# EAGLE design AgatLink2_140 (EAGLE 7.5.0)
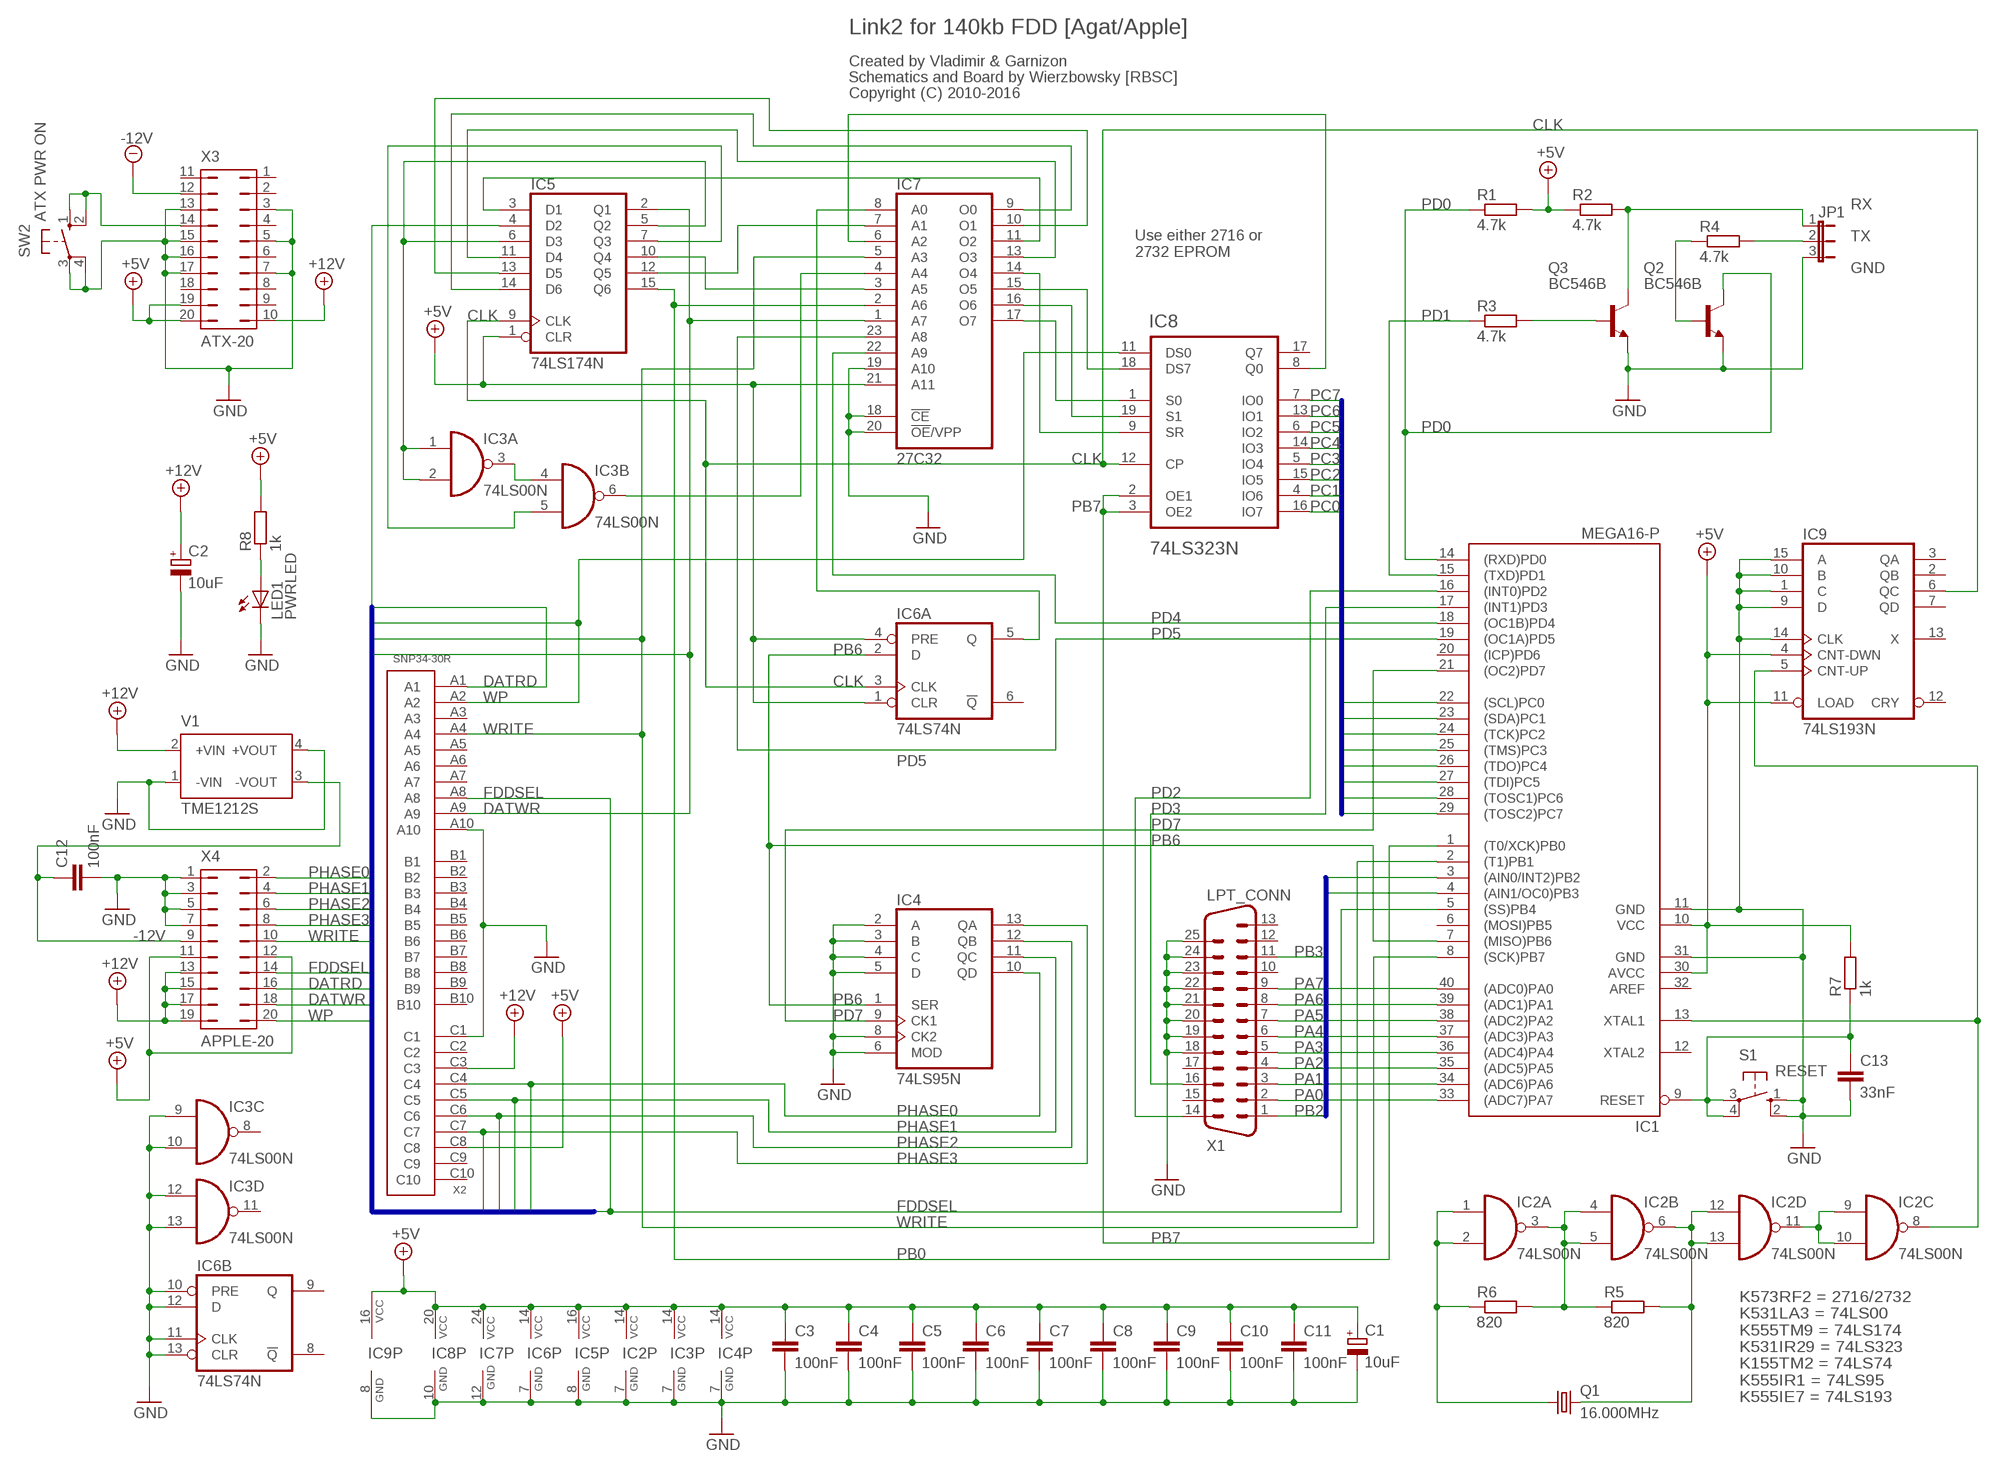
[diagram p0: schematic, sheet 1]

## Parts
C1  10uF  CPOL-EUE2-5  [E2-5]
C2  10uF  CPOL-EUE2-5  [E2-5]
C3  100nF  C-EU050-025X075  [C050-025X075]
C4  100nF  C-EU050-025X075  [C050-025X075]
C5  100nF  C-EU050-025X075  [C050-025X075]
C6  100nF  C-EU050-025X075  [C050-025X075]
C7  100nF  C-EU050-025X075  [C050-025X075]
C8  100nF  C-EU050-025X075  [C050-025X075]
C9  100nF  C-EU050-025X075  [C050-025X075]
C10  100nF  C-EU050-025X075  [C050-025X075]
C11  100nF  C-EU050-025X075  [C050-025X075]
C12  100nF  C-EU050-025X075  [C050-025X075]
C13  33nF  C-EU025-025X050  [C025-025X050]
IC1  MEGA16-P  [DIL40]
IC2  74LS00N  [DIL14]
IC3  74LS00N  [DIL14]
IC4  74LS95N  [DIL14]
IC5  74LS174N  [DIL16]
IC6  74LS74N  [DIL14]
IC7  27C32  2732  [DIL24]
IC8  74LS323N  [DIL20]
IC9  74LS193N  [DIL16]
JP1  JP2E  [JP2]
LED1  PWRLED  LED3MM  [LED3MM]
Q1  16.000MHz  CRYSTALHC49S  [HC49/S]
Q2  BC546B  [TO92-EBC]
Q3  BC546B  [TO92-EBC]
R1  4.7k  R-EU_0204/7  [0204/7]
R2  4.7k  R-EU_0204/7  [0204/7]
R3  4.7k  R-EU_0204/7  [0204/7]
R4  4.7k  R-EU_0204/7  [0204/7]
R5  820  R-EU_0204/7  [0204/7]
R6  820  R-EU_0204/7  [0204/7]
R7  1k  R-EU_0204/7  [0204/7]
R8  1k  R-EU_0204/7  [0204/7]
S1  RESET  10-XX  [B3F-10XX]
SW2  ATX PWR ON  10-XX  [B3F-10XX]
V1  TME1212S  [TME]
X1  LPT_CONN  M25HP  [M25HP]
X2  SNP34-30R  [SNP34-30R]
X3  ATX-20  [ATX-20]
X4  APPLE-20  [APPLE-20]

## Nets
+5V: C1.+ C3.1 C4.1 C5.1 C6.1 C7.1 C8.1 C9.1 C10.1 C11.1 IC1.10(VCC) IC1.30(AVCC) IC2.14(P:VCC) IC3.14(P:VCC) IC4.14(VCC) IC5.1(CLR) IC5.16(VCC) IC6.1(A:CLR) IC6.4(A:PRE) IC6.14(P:VCC) IC7.21(A11) IC7.24(VCC) IC8.20(VCC) IC9.4(CNT-DWN) IC9.11(LOAD) IC9.16(VCC) R1.2 R2.1 R7.2 R8.2 X2.C8 X3.19 X3.20 X4.11 X4.12
+12V: C2.+ V1.2(+VIN) X2.C3 X3.10 X4.13 X4.15 X4.17 X4.19
-12V: C12.1 V1.3(-VOUT) X3.12 X4.9
CLK: IC5.9(CLK) IC6.3(A:CLK) IC8.12(CP) IC9.6(QC)
DATRD: IC5.4(D2) X2.A1 X4.16
DATWR: IC5.2(Q1) IC7.1(A7) X2.A9 X4.18
FDDSEL: IC1.5((SS)PB4) X2.A8 X4.14
GND: C1.- C2.- C3.2 C4.2 C5.2 C6.2 C7.2 C8.2 C9.2 C10.2 C11.2 C12.2 C13.2 IC1.11(GND) IC1.31(GND) IC2.7(P:GND) IC3.7(P:GND) IC3.9(C:I0) IC3.10(C:I1) IC3.12(D:I0) IC3.13(D:I1) IC4.2(A) IC4.3(B) IC4.4(C) IC4.5(D) IC4.6(MOD) IC4.7(GND) IC4.8(CK2) IC5.8(GND) IC6.7(P:GND) IC6.10(B:PRE) IC6.11(B:CLK) IC6.12(B:D) IC6.13(B:CLR) IC7.12(GND) IC7.18(!CE) IC7.19(A10) IC7.20(!OE!/VPP) IC8.10(GND) IC9.1(C) IC9.8(GND) IC9.9(D) IC9.10(B) IC9.14(CLK) IC9.15(A) JP1.3 LED1.K(C) Q2.E Q3.E S1.1(S) S1.2(S1) SW2.3(P) SW2.4(P1) V1.1(-VIN) V1.4(+VOUT) X1.18 X1.19 X1.20 X1.21 X1.22 X1.23 X1.24 X1.25 X2.A10 X2.C1 X3.3 X3.5 X3.7 X3.13 X3.15 X3.16 X3.17 X4.1 X4.3 X4.5 X4.7
N$1: IC2.1(A:I0) IC2.2(A:I1) Q1.1 R6.1
N$2: IC2.3(A:O) IC2.4(B:I0) IC2.5(B:I1) R5.1 R6.2
N$3: IC1.13(XTAL1) IC2.8(C:O) IC9.5(CNT-UP)
N$4: SW2.1(S) SW2.2(S1) X3.14
N$6: IC2.6(B:O) IC2.12(D:I0) IC2.13(D:I1) Q1.2 R5.2
N$8: IC2.9(C:I0) IC2.10(C:I1) IC2.11(D:O)
N$11: C13.1 IC1.9(RESET) R7.1 S1.3(P) S1.4(P1)
N$12: JP1.1 Q3.C R2.2
N$13: Q3.B R3.2
N$15: JP1.2 R4.2
N$16: Q2.B R4.1
N$17: LED1.A R8.1
N$19: IC3.3(A:O) IC3.4(B:I0)
N$20: IC3.1(A:I0) IC3.2(A:I1) IC5.5(Q2) IC5.6(D3)
N$22: IC3.5(B:I1) IC5.7(Q3)
N$23: IC3.6(B:O) IC7.4(A4)
N$24: IC6.5(A:Q) IC7.8(A0)
N$27: IC7.14(O4) IC8.9(SR)
N$28: IC7.17(O7) IC8.1(S0)
N$29: IC7.16(O6) IC8.19(S1)
N$30: IC7.15(O5) IC8.18(DS7)
N$35: IC5.3(D1) IC7.11(O2)
N$36: IC5.11(D4) IC7.13(O3)
N$37: IC5.14(D6) IC7.9(O0)
N$38: IC5.13(D5) IC7.10(O1)
N$39: IC5.10(Q4) IC7.3(A5)
N$40: IC5.12(Q5) IC7.7(A1)
N$41: IC7.6(A2) IC8.8(Q0)
PA0: IC1.40((ADC0)PA0) X1.2
PA1: IC1.39((ADC1)PA1) X1.3
PA2: IC1.38((ADC2)PA2) X1.4
PA3: IC1.37((ADC3)PA3) X1.5
PA4: IC1.36((ADC4)PA4) X1.6
PA5: IC1.35((ADC5)PA5) X1.7
PA6: IC1.34((ADC6)PA6) X1.8
PA7: IC1.33((ADC7)PA7) X1.9
PB0: IC1.1((T0/XCK)PB0) IC5.15(Q6) IC7.2(A6)
PB2: IC1.3((AIN0/INT2)PB2) X1.1
PB3: IC1.4((AIN1/OC0)PB3) X1.11
PB6: IC1.7((MISO)PB6) IC4.1(SER) IC6.2(A:D)
PB7: IC1.8((SCK)PB7) IC8.2(OE1) IC8.3(OE2)
PC0: IC1.22((SCL)PC0) IC8.16(IO7)
PC1: IC1.23((SDA)PC1) IC8.4(IO6)
PC2: IC1.24((TCK)PC2) IC8.15(IO5)
PC3: IC1.25((TMS)PC3) IC8.5(IO4)
PC4: IC1.26((TDO)PC4) IC8.14(IO3)
PC5: IC1.27((TDI)PC5) IC8.6(IO2)
PC6: IC1.28((TOSC1)PC6) IC8.13(IO1)
PC7: IC1.29((TOSC2)PC7) IC8.7(IO0)
PD0: IC1.14((RXD)PD0) Q2.C R1.1
PD1: IC1.15((TXD)PD1) R3.1
PD2: IC1.16((INT0)PD2) X1.14
PD3: IC1.17((INT1)PD3) X1.16
PD4: IC1.18((OC1B)PD4) IC7.22(A9)
PD5: IC1.19((OC1A)PD5) IC7.23(A8)
PD7: IC1.21((OC2)PD7) IC4.9(CK1)
PHASE0: IC4.10(QD) X2.C4 X4.2
PHASE1: IC4.11(QC) X2.C5 X4.4
PHASE2: IC4.12(QB) X2.C6 X4.6
PHASE3: IC4.13(QA) X2.C7 X4.8
WP: IC8.11(DS0) X2.A2 X4.20
WRITE: IC1.2((T1)PB1) IC7.5(A3) X2.A4 X4.10
Unconnected: IC1.6((MOSI)PB5) IC1.12(XTAL2) IC1.20((ICP)PD6) IC1.32(AREF) IC3.8(C:O) IC3.11(D:O) IC6.6(A:!Q) IC6.8(B:!Q) IC6.9(B:Q) IC8.17(Q7) IC9.2(QB) IC9.3(QA) IC9.7(QD) IC9.12(CRY) IC9.13(X) X1.10 X1.12 X1.13 X1.15 X1.17 X2.A3 X2.A5 X2.A6 X2.A7 X2.B1 X2.B2 X2.B3 X2.B4 X2.B5 X2.B6 X2.B7 X2.B8 X2.B9 X2.B10 X2.C2 X2.C9 X2.C10 X3.1 X3.2 X3.4 X3.6 X3.8 X3.9 X3.11 X3.18

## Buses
PA0,PA1,PA2,PA3,PA4,PA5,PA6,PA7,PB2,PB3
PC0,PC1,PC2,PC3,PC4,PC5,PC6,PC7
DATRD,WP,WRITE,FDDSEL,DATWR,PHASE0,PHASE1,PHASE2,PHASE3

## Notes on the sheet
- Link2 for 140kb FDD [Agat/Apple]
- Created by Vladimir & Garnizon
- Schematics and Board by Wierzbowsky [RBSC]
- Copyright (C) 2010-2016
- RX
- TX
- Use either 2716 or
  2732 EPROM
- GND
- K573RF2 = 2716/2732
  K531LA3 = 74LS00
  K555TM9 = 74LS174
  K531IR29 = 74LS323
  K155TM2 = 74LS74
  K555IR1 = 74LS95
  K555IE7 = 74LS193

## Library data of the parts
C1 C2 = rcl:CPOL-EU: POLARIZED CAPACITOR, European symbol
C3-C13 = rcl:C-EU: CAPACITOR, European symbol
IC1 = atmel:MEGA16-P: MICROCONTROLLER 16 Kbytes FLASH 1 kbytes SRAM 512 bytes EEPROM USART 8-channel 10 bit ADC Source: avr.lbr; MPN: ATMEGA16-16PU; OC_FARNELL: 9171142; OC_NEWARK: 01M6885
IC2 IC3 = 74xx-eu:74*00: Quad 2-input NAND gate
IC4 = 74xx-eu:74*95: 4-bit parallel access SHIFT REGISTER
IC5 = 74xx-eu:74*174: Hex D type FLIP FLOP, clear
IC6 = 74xx-eu:74*74: Dual D type positive edge triggered FLIP FLOP, preset and clear
IC7 = memory:2732: MEMORY
IC8 = 74LS323:74LS323N: 74LS323
IC9 = 0RB_TTL:74*193: Synchronous UP/DOWN COUNTER
JP1 = jumper:JP2E: JUMPER
LED1 = led:LED: LED
Q1 = crystal:CRYSTAL: CRYSTAL; OC_FARNELL: 1667008; OC_NEWARK: unknown
Q2 Q3 = transistor-npn:BC546*: NPN Transistor
R1-R8 = resistor:R-EU_: RESISTOR, European symbol
S1 SW2 = switch-omron:10-XX: OMRON SWITCH; MPN: B3F-1000; OC_FARNELL: 176432; OC_NEWARK: 36M3542
V1 = traco-electronic:TME?*: DC/DC Converter TME Series 1 Watt Source: www.tracopower.com .. tme.pdf; MPN: TME 1212S; OC_FARNELL: 1007545; OC_NEWARK: 51R5327
X1 = con-subd:M25: SUB-D; OC_FARNELL: unknown; OC_NEWARK: unknown
X2 = snp34-30:SNP34-30R
X3 = atx_conn:ATX-20: ATX PC-Motherboard Power connector
X4 = apple_fdd_conn:APPLE-20: Apple Disk II connector

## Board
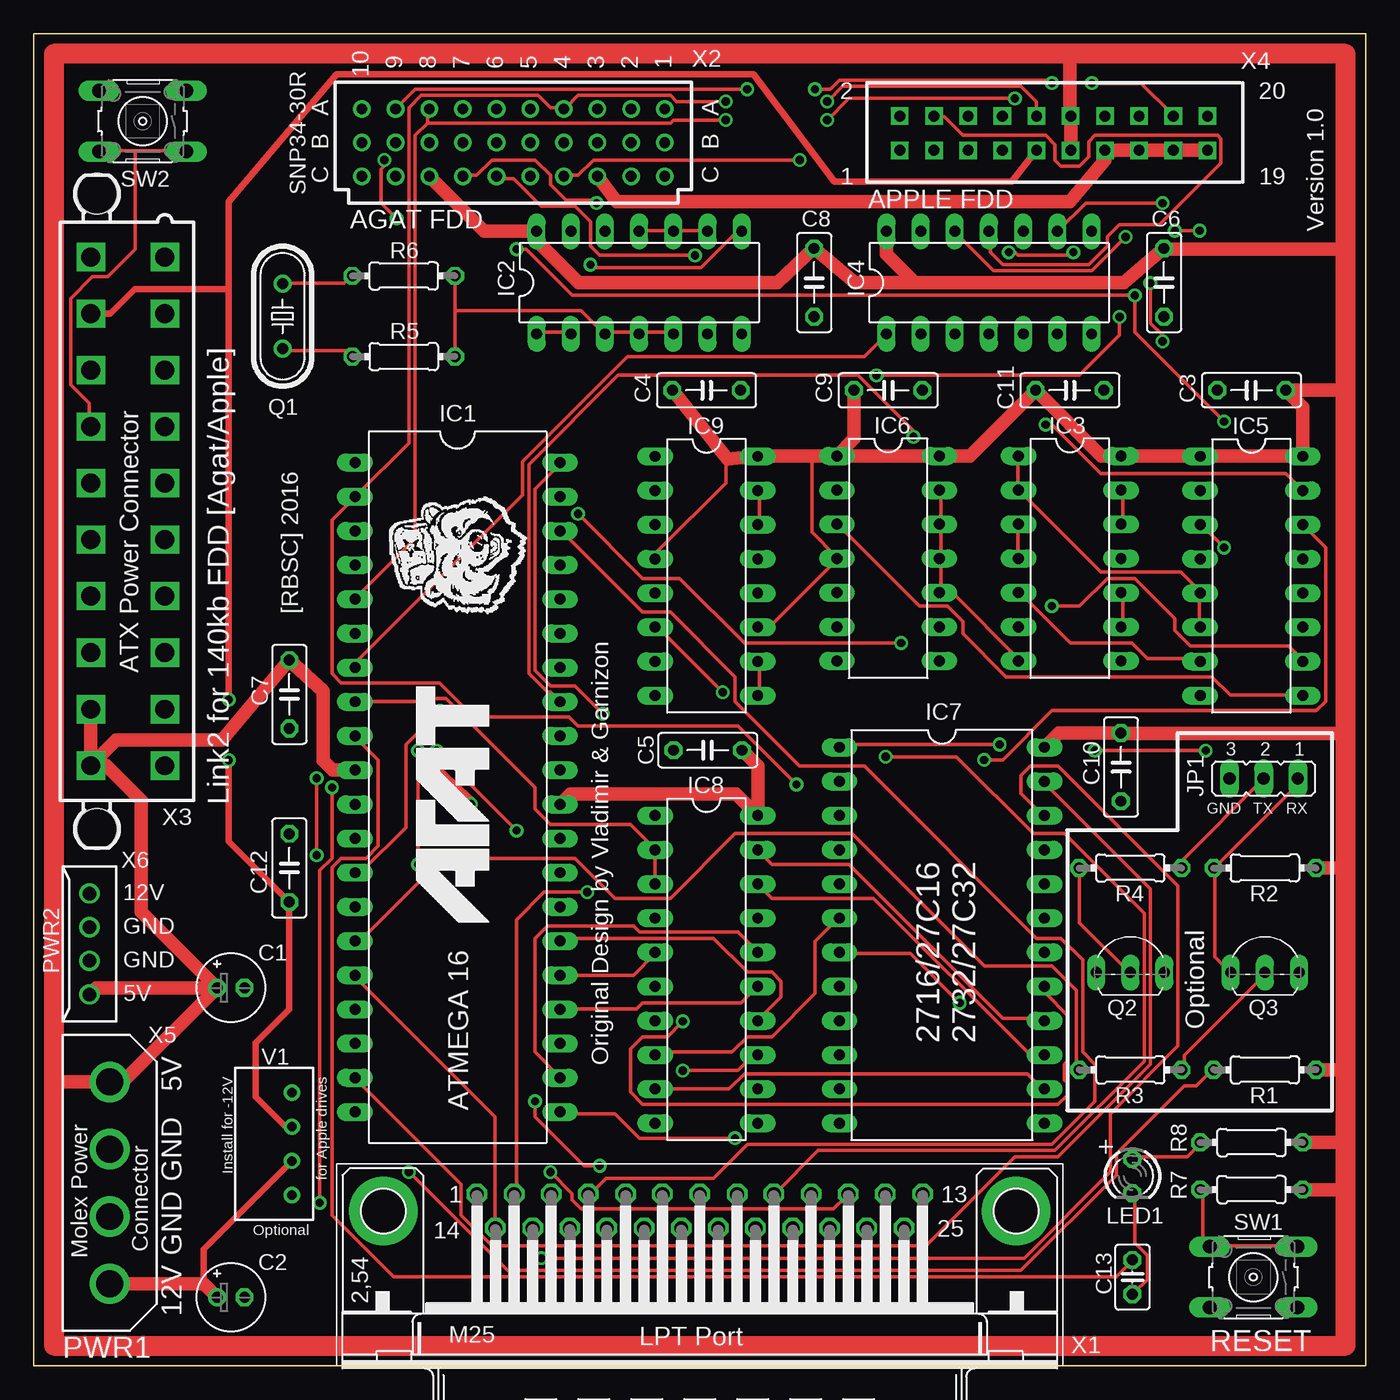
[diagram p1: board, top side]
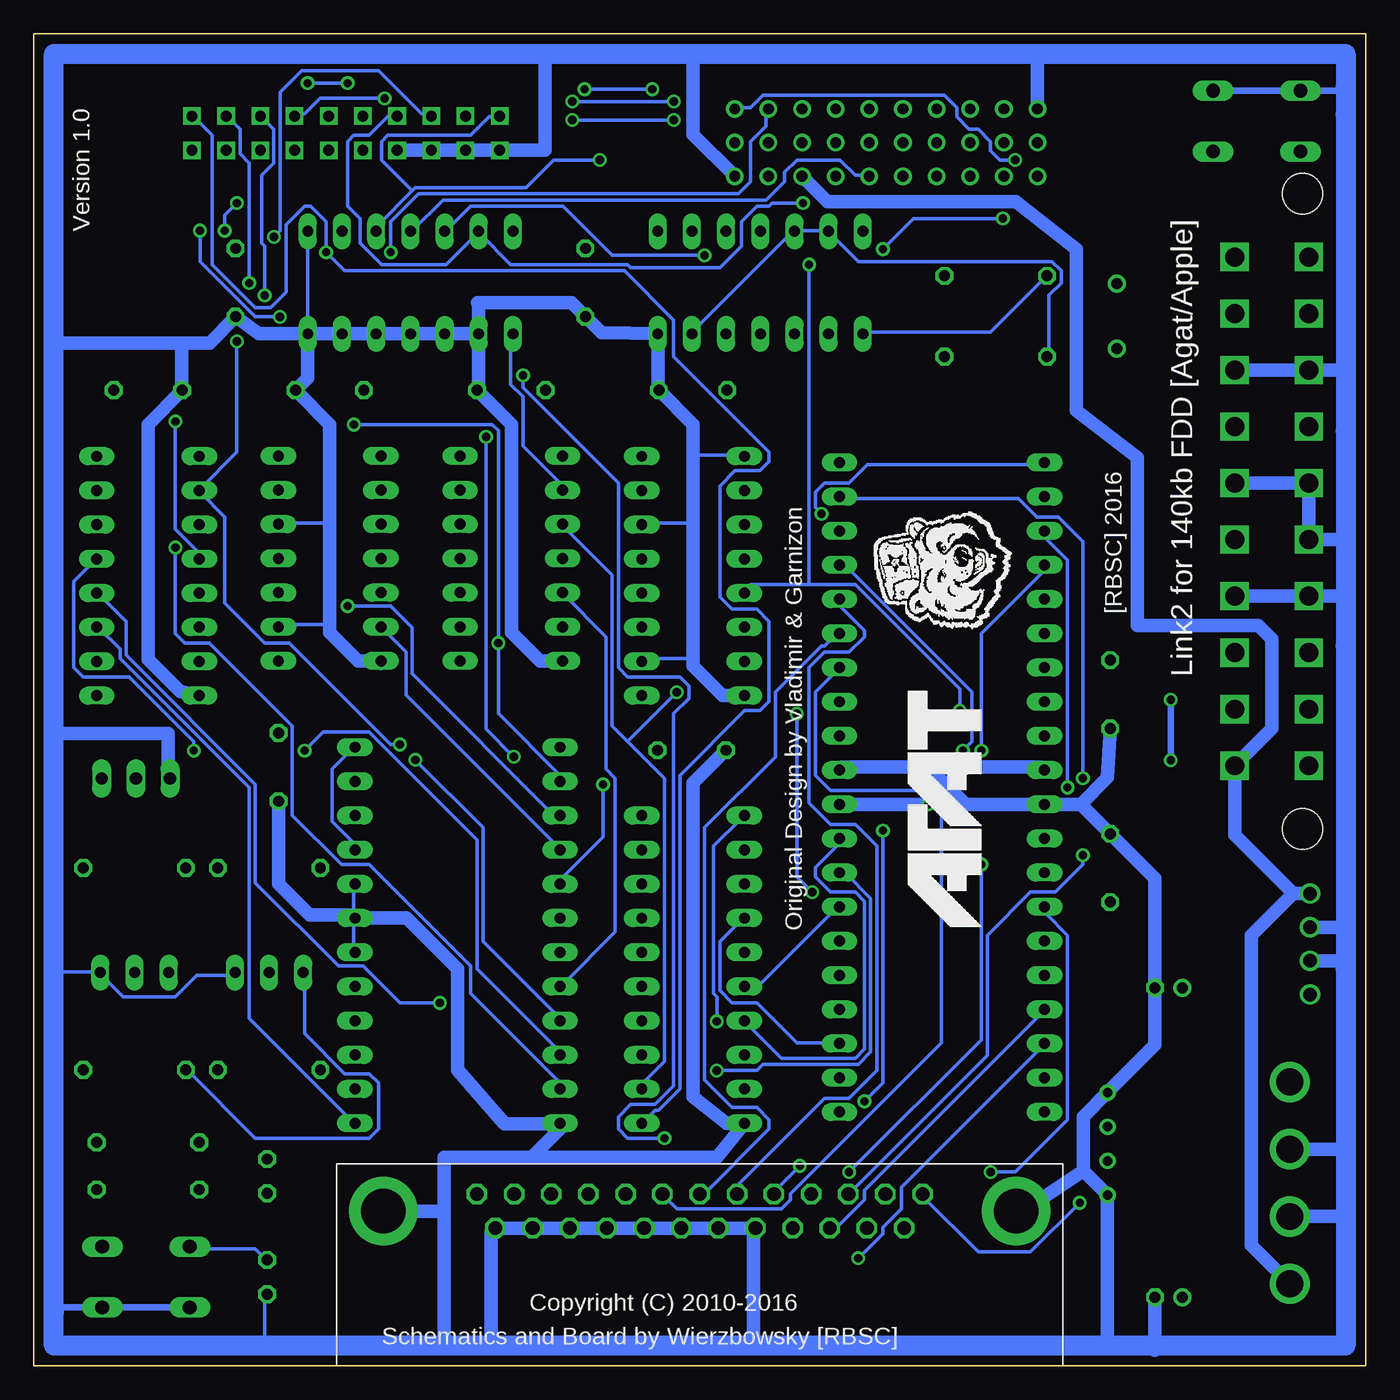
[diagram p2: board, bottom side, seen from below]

Size 99 x 99 mm. Coordinates in mm from the lower left corner, seen from the top.
Outline: 0,0 0,99 99,99 99,0 0,0
Copper layers (1*16): Top 0.035mm / dielectric 1.5mm / Bottom 0.035mm
Design rules "default *": minimum track width 10mil, minimum drill 24mil, track to track 8mil, track to pad 8mil, pad to pad 8mil, via to via 8mil, smd to smd 8mil, copper to edge 40mil, drill to drill 8mil, minimum pad ring 10mil, minimum via ring 8mil, stop-mask expansion 4mil, vias tented up to drill 24mil, thermal gap 10mil

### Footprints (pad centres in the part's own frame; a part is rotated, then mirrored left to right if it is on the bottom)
E2-5 = drill 0.813 pad 1.27: + -1.016,0 | drill 0.813 pad 1.27 octagon: - 1.016,0
C050-025X075 = drill 0.813 octagon: 1 -2.54,0; 2 2.54,0
C025-025X050 = drill 0.813 octagon: 1 -1.27,0; 2 1.27,0
DIL40 = drill 0.813 long: 1 -24.13,-7.62; 2 -21.59,-7.62; 3 -19.05,-7.62; 4 -16.51,-7.62; 5 -13.97,-7.62; 6 -11.43,-7.62; 7 -8.89,-7.62; 8 -6.35,-7.62; 9 -3.81,-7.62; 10 -1.27,-7.62; 11 1.27,-7.62; 12 3.81,-7.62; 13 6.35,-7.62; 14 8.89,-7.62; 15 11.43,-7.62; 16 13.97,-7.62; 17 16.51,-7.62; 18 19.05,-7.62; 19 21.59,-7.62; 20 24.13,-7.62; 21 24.13,7.62; 22 21.59,7.62; 23 19.05,7.62; 24 16.51,7.62; 25 13.97,7.62; 26 11.43,7.62; 27 8.89,7.62; 28 6.35,7.62; 29 3.81,7.62; 30 1.27,7.62; 31 -1.27,7.62; 32 -3.81,7.62; 33 -6.35,7.62; 34 -8.89,7.62; 35 -11.43,7.62; 36 -13.97,7.62; 37 -16.51,7.62; 38 -19.05,7.62; 39 -21.59,7.62; 40 -24.13,7.62
DIL14 = drill 0.813 long: 1 -7.62,-3.81; 2 -5.08,-3.81; 3 -2.54,-3.81; 4 0,-3.81; 5 2.54,-3.81; 6 5.08,-3.81; 7 7.62,-3.81; 8 7.62,3.81; 9 5.08,3.81; 10 2.54,3.81; 11 0,3.81; 12 -2.54,3.81; 13 -5.08,3.81; 14 -7.62,3.81
DIL16 = drill 0.813 long: 1 -8.89,-3.81; 2 -6.35,-3.81; 3 -3.81,-3.81; 4 -1.27,-3.81; 5 1.27,-3.81; 6 3.81,-3.81; 7 6.35,-3.81; 8 8.89,-3.81; 9 8.89,3.81; 10 6.35,3.81; 11 3.81,3.81; 12 1.27,3.81; 13 -1.27,3.81; 14 -3.81,3.81; 15 -6.35,3.81; 16 -8.89,3.81
DIL24 = drill 0.813 long: 1 -13.97,-7.62; 2 -11.43,-7.62; 3 -8.89,-7.62; 4 -6.35,-7.62; 5 -3.81,-7.62; 6 -1.27,-7.62; 7 1.27,-7.62; 8 3.81,-7.62; 9 6.35,-7.62; 10 8.89,-7.62; 11 11.43,-7.62; 12 13.97,-7.62; 13 13.97,7.62; 14 11.43,7.62; 15 8.89,7.62; 16 6.35,7.62; 17 3.81,7.62; 18 1.27,7.62; 19 -1.27,7.62; 20 -3.81,7.62; 21 -6.35,7.62; 22 -8.89,7.62; 23 -11.43,7.62; 24 -13.97,7.62
DIL20 = drill 0.813 long: 1 -8.89,-3.81; 2 -6.35,-3.81; 3 -3.81,-3.81; 4 -1.27,-3.81; 5 1.27,-3.81; 6 3.81,-3.81; 7 6.35,-3.81; 8 8.89,-3.81; 9 11.43,-3.81; 10 13.97,-3.81; 11 13.97,3.81; 12 11.43,3.81; 13 8.89,3.81; 14 6.35,3.81; 15 3.81,3.81; 16 1.27,3.81; 17 -1.27,3.81; 18 -3.81,3.81; 19 -6.35,3.81; 20 -8.89,3.81
JP2 = drill 0.914 long: 1 -2.54,0; 2 0,0; 3 2.54,0
LED3MM = drill 0.813 octagon: A -1.27,0; K 1.27,0
HC49/S = drill 0.813: 1 -2.413,0; 2 2.413,0
TO92-EBC = drill 0.813 long: B 0,-1.27; C -2.54,-1.27; E 2.54,-1.27
0204/7 = drill 0.813 octagon: 1 -3.81,0; 2 3.81,0
B3F-10XX = drill 1.016 long: 1 -3.251,2.261; 2 3.251,2.261; 3 -3.251,-2.261; 4 3.251,-2.261
TME = drill 0.7 pad 1.1: 1 -3.81,0; 2 -1.27,0; 3 1.27,0; 4 3.81,0
M25HP = drill 1.016 octagon: 1 -16.561,1.27; 2 -13.792,1.27; 3 -11.049,1.27; 4 -8.28,1.27; 5 -5.512,1.27; 6 -2.769,1.27; 7 0,1.27; 8 2.769,1.27; 9 5.512,1.27; 10 8.28,1.27; 11 11.049,1.27; 12 13.792,1.27; 13 16.561,1.27; 14 -15.189,-1.27; 15 -12.421,-1.27; 16 -9.652,-1.27; 17 -6.909,-1.27; 18 -4.14,-1.27; 19 -1.372,-1.27; 20 1.372,-1.27; 21 4.14,-1.27; 22 6.909,-1.27; 23 9.652,-1.27; 24 12.421,-1.27; 25 15.189,-1.27 | drill 3.302 pad 5.08: G1 -23.52,0; G2 23.52,0
SNP34-30R = drill 0.8: A1 -2,2; A2 -2,4.5; A3 -2,7; A4 -2,9.5; A5 -2,12; A6 -2,14.5; A7 -2,17; A8 -2,19.5; A9 -2,22; A10 -2,24.5; B1 -4.5,2; B2 -4.5,4.5; B3 -4.5,7; B4 -4.5,9.5; B5 -4.5,12; B6 -4.5,14.5; B7 -4.5,17; B8 -4.5,19.5; B9 -4.5,22; B10 -4.5,24.5; C1 -7,2; C2 -7,4.5; C3 -7,7; C4 -7,9.5; C5 -7,12; C6 -7,14.5; C7 -7,17; C8 -7,19.5; C9 -7,22; C10 -7,24.5
ATX-20 = drill 1.4 square: 1 18.9,-2.75; 2 14.7,-2.75; 3 10.5,-2.75; 4 6.3,-2.75; 5 2.1,-2.75; 6 -2.1,-2.75; 7 -6.3,-2.75; 8 -10.5,-2.75; 9 -14.7,-2.75; 10 -18.9,-2.75; 11 18.9,2.75; 12 14.7,2.75; 13 10.5,2.75; 14 6.3,2.75; 15 2.1,2.75; 16 -2.1,2.75; 17 -6.3,2.75; 18 -10.5,2.75; 19 -14.7,2.75; 20 -18.9,2.75 | hole 3: 23.6,2.29; -23.6,2.29
APPLE-20 = drill 0.8 square: 1 -11.43,-1.27; 2 -11.43,1.27; 3 -8.89,-1.27; 4 -8.89,1.27; 5 -6.35,-1.27; 6 -6.35,1.27; 7 -3.81,-1.27; 8 -3.81,1.27; 9 -1.27,-1.27; 10 -1.27,1.27; 11 1.27,-1.27; 12 1.27,1.27; 13 3.81,-1.27; 14 3.81,1.27; 15 6.35,-1.27; 16 6.35,1.27; 17 8.89,-1.27; 18 8.89,1.27; 19 11.43,-1.27; 20 11.43,1.27

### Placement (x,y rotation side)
C1  14.65,28.1 0 top
C2  14.65,5.1 0 top
C3  90.5,72.5 180 top
C4  50,72.5 0 top
C5  50.1,45.75 180 top
C6  84,80.5 270 top
C7  19,49.9 270 top
C8  58,80.5 270 top
C9  63.5,72.5 0 top
C10  80.8,44.5 270 top
C11  77,72.5 0 top
C12  19,37 90 top
C13  81.65,6.6 270 top
IC1  31.5,43 270 top
IC2  45,80.5 0 top
IC3  77,60 270 top
IC4  71,80.5 0 top
IC5  90.5,58.7 270 top
IC6  63.5,60 270 top
IC7  67.5,32 270 top
IC8  50,32 270 top
IC9  50,58.7 270 top
JP1  91.4,43.65 180 top
LED1  81.65,14.1 270 top
Q1  18.5,78 270 top
Q2  81.5,30.5 0 top
Q3  91.5,30.5 0 top
R1  91.5,22 0 top
R2  91.5,37 180 top
R3  81.5,22 0 top
R4  81.5,37 0 top
R5  27.5,75 180 top
R6  27.5,81 0 top
R7  90.5,13.1 0 top
R8  90.5,16.6 0 top
S1  90.65,6.6 180 top
SW2  8.1,92.5 180 top
V1  19.2,16.5 90 top
X1  49.5,11.5 0 top
X2  48.9,95.4 90 top
X3  7,63.5 90 top
X4  75.8,91.6 0 top

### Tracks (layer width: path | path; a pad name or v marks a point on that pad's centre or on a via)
+5V  (via drill 0.61, 1, 2)
  Top 0.254: IC9.11 53.95,55.09 54.86,55.09 59.66,59.89 IC6.4 59.66,60.12 57.84,61.95 57.84,67.62 | IC9.4 46.41,60.12 46.41,60.58 51.44,65.61 51.44,66.98 51.57,67.39
  Top 1: IC1.10 22.23,44.27 21.5,45 21.5,50.14 C7.1 14,46.5 6.15,46.5 X3.20 | R2.1 97.5,37 | IC6.1 57.84,67.62 54.04,67.62 IC9.16 51.57,67.39 C4.1 | IC6.1 60.96,68.89 C9.1 | 77,97.5 77,92.94 X4.12 X4.11 | 65.5,80.5 61.04,80.5 C8.1 55.26,80.5 40.5,80.5 37.38,83.62 IC2.14 33.49,84.31 X2.C8 | 65.5,80.5 81.01,80.5 C6.1 83.99,83 97.5,83 | 93,72.5 C3.1 | C3.1 97.5,72.5 | IC1.30 39.89,42.5 52.2,42.5 IC8.20 53.81,44.58 C5.1 | R1.2 97.5,22 | R8.2 97.4,16.6 97.5,16 | R7.2 97.4,13.1 97.5,12.5 | IC6.1 IC6.14 69.58,67.62 C11.1 79.34,67.62 IC3.14 86.42,67.62 IC5.1 IC5.16 94.31,71.23 C3.1 | IC4.14 63.38,82.62 65.5,80.5 | v29.5,44.5 v32.5,41.73 | 97.5,47 80.84,47 C10.1 76.19,47.04 IC7.24 | 1.5,21 1.5,21.1 v5.65,21.1 6.64,21.1 C1.+ | 1.6,27.6 1.5,27.5 | X3.20 5.4,44.6 8,42 8,33.73 C1.+ | X3.20 X3.19 | v4.15,27.6 4.65,28.1 C1.+
  Top 1.5: 1.5,1.5 97.5,1.5 97.5,12.5 97.5,16 97.5,22 97.5,37 97.5,47 97.5,72.5 97.5,83 97.5,97.5 77,97.5 1.5,97.5 1.5,27.5 1.5,21 1.5,1.5
  Bottom 0.254: IC7.21 75.21,38.41 75.21,38.86 76.81,40.46 76.81,44.35 75.21,45.95 IC7.24
  Bottom 1: IC1.10 24.15,44.5 v29.5,44.5 | IC1.30 v32.5,41.73
+12V  (via drill 1, 2)
  Top 0.5: 12.63,6.1 12.63,8.66 V1.2
  Top 1: X2.C3 43.3,86.5 77,86.5 79.61,89.61 X4.13 X4.15 X4.17 X4.19 | v5.65,6.1 12.63,6.1 C2.+
  Bottom 1: X2.C3 40,86.5 26,86.5 21.5,83 21.5,71 17,67.5 17,55 8,55 7,54 7,47.35 X3.10 9.75,39.44 5.4,35.1 | v4.15,35.1 5.4,35.1 | 5.4,35.1 8.5,32 8.5,8.95 v5.65,6.1
-12V  (via drill 0.61)
  Top 0.5: V1.3 18.73,17.77 16.5,20 16.5,24 19,26.5 C12.1 14.5,38.96 v14.5,45 | v14.5,49.5 14.5,80 | 14.5,80 14.5,86.5 22.5,96 53.5,96 59.5,88 72.7,88 X4.9 | X3.12 5.7,78.2 7.5,80 14.5,80
  Bottom 0.5: v14.5,45 v14.5,49.5
CLK  (via drill 0.61)
  Top 0.254: IC5.9 94.18,49.84 88.92,49.84 87.55,51.21 72.24,51.21 69.04,54.41 69.04,55.32 67.89,56.46 65.84,56.46 59.89,62.41 IC6.3 | v51.21,50.06 46.41,54.86 IC9.6
  Bottom 0.254: 54.86,46.41 56.01,47.55 56.01,58.75 59.66,62.41 IC6.3 | 54.86,46.41 52.12,43.66 52.12,22.63 53.72,21.03 53.72,20.57 IC8.12 | 54.86,46.41 v51.21,50.06
DATRD  (via drill 0.61)
  Top 0.254: v26.06,89.61 26.06,89.15 25.83,88.92 25.83,86.41 v26.98,85.27 | v35.89,82.98 36.58,82.98 40.01,79.55 v81.84,79.55 81.84,76.81 v88.47,70.18
  Bottom 0.254: v26.06,89.61 27.2,89.61 27.89,90.3 27.89,90.98 28.8,91.9 29.49,91.9 30.4,92.81 30.4,93.5 31.32,94.41 44.81,94.41 45.72,93.5 46.86,93.5 X2.A1 | v26.98,85.27 33.6,85.27 v35.89,82.98 | v81.84,79.55 81.84,83.21 82.07,83.44 82.07,88.47 81.15,89.38 81.15,91.9 82.07,92.81 X4.16 | v88.47,70.18 88.47,62.18 86.87,60.58 86.87,60.12 IC5.4
DATWR  (via drill 0.61)
  Top 0.254: v71.78,46.18 59.89,46.18 IC7.1 | v53.03,94.87 28.35,94.87 26.98,93.5 X2.A9 | v58.06,94.87 59.21,94.87 59.89,95.56 75.44,95.56 v75.67,95.33 | v78.64,95.33 82.3,95.33 84.58,93.04 X4.18 | v83.9,76.12 83.9,76.58 82.98,77.5 v82.98,80.47
  Bottom 0.254: v71.78,46.18 72.47,46.18 80.01,53.72 81.84,53.72 84.81,56.69 84.81,63.09 86.64,64.92 IC5.2 86.64,65.15 83.9,67.89 v83.9,76.12 | v58.06,94.87 v53.03,94.87 | v78.64,95.33 v75.67,95.33 | v82.98,80.47 82.98,89.38 83.67,90.07 83.67,91.9 84.58,92.81 X4.18
FDDSEL  (via drill 0.61)
  Top 0.254: 29.26,92.35 29.26,93.27 X2.A8 | 29.26,92.35 28.35,91.44 28.35,61.49 24,57.15 IC1.5 | v72.92,94.18 60.58,94.18 v58.98,92.58 | v51.44,92.58 47.55,92.58 47.32,92.35 29.26,92.35
  Bottom 0.254: v72.92,94.18 77.72,94.18 78.87,93.04 79.55,93.04 X4.14 | v51.44,92.58 v58.98,92.58
GND  (via drill 1, 2)
  Top 0.254: IC6.13 67.44,64.92 67.44,62.64 IC6.12 67.44,62.41 67.44,60.12 IC6.11 67.44,59.89 67.44,57.61 IC6.10 67.44,57.38 68.35,57.38 73.15,52.58 IC3.7 | IC3.12 80.92,62.64 80.92,64.92 IC3.13 | IC3.9 80.92,55.09 80.92,57.38 IC3.10 | IC9.14 53.95,62.64 53.95,64.92 IC9.15 | IC9.9 53.95,49.84 53.95,52.35 IC9.10 | LED1.K 81.84,12.8 81.84,9.14 82.75,8.23 82.75,6.4 81.84,5.49 C13.2
  Bottom 0.254: C3.2 88.01,72.69 88,72.69 | Q2.E 84.12,29.03 86.87,29.03 88.47,27.43 92.35,27.43 93.95,29.03 Q3.E 94.18,29.26 97.5,29.26 | 81.84,1.5 81.84,5.26 C13.2 | IC7.18 75.21,30.86 75.21,32.92 IC7.19 75.21,33.83 75.21,35.66 IC7.20 | 50,67.67 46.41,67.67 IC9.1 | IC4.8 78.64,84.12 78.64,77.04 IC4.7 | 50,52.58 53.72,52.58 IC9.10 | 50,62.64 53.72,62.64 IC9.14 | 77,55.09 80.7,55.09 IC3.9 | 77,62.64 80.7,62.64 IC3.12
  Bottom 0.5: SW2.3 SW2.4 1.74,94.76 1.5,95 | 1.24,94.76 1.5,93 | S1.2 S1.1 97.16,4.34 97.5,4
  Bottom 1: C2.- 15.67,1.17 15.5,1.5 | 19.5,1.5 19.2,1.3 V1.1 21,14.5 | 21,14.5 21,18.51 V1.4 15.67,23.84 C1.- 15.67,36.21 C12.2 21.19,41.73 | 21.19,41.73 IC1.11 29.73,41.73 32.5,44.5 38.89,44.5 IC1.31 | C7.2 19.2,43.72 21.19,41.73 | X3.7 X3.17 1.7,57.2 1.5,57 | 1.7,53.2 1.5,53 1.5,53.5 | X3.5 X3.15 X3.16 1.6,61.4 1.5,61.5 | 1.5,70 1.5,69.5 | X3.3 X3.13 1.5,74 | X2.A10 24.4,97.4 24.5,97.5 | X1.18 45.5,10.09 | 45.5,10.09 45.5,1.5 | 65,1.5 65,9.92 X1.25 X1.24 X1.23 X1.22 X1.21 X1.20 X1.19 45.64,10.23 45.5,10.09 | 73.19,52.19 IC3.7 74.88,52.38 77,54.5 77,55.09 77,62.64 77,69.96 C11.2 78.62,73.42 IC4.7 | 62,15.5 48.22,15.5 IC8.10 47.53,18.03 50,20 50,43.31 C5.2 | 62,15.5 68.5,15.5 68.5,11.5 | 68.5,11.5 68.5,1.5 69,1.5 | X4.7 X4.5 X4.3 X4.1 61,90.33 61,97.5 | IC2.7 56.7,76.77 56.81,76.77 C8.2 59.04,79 66,79 65.92,78.92 IC4.2 | 88,76 85.91,76 C6.2 82.28,76.69 IC4.7 | 88,76 97.5,76 | IC2.7 52.54,76.61 | 93.9,1.6 94,1.5 | C10.2 80.8,35.8 78.5,33.5 75.35,33.5 IC7.19 71.27,33.27 67.5,29.5 67.5,22 64,18 60.35,18 IC7.12 59.88,17.62 62,15.5 | C3.2 90.5,69.96 90.5,52.5 88.11,50.11 IC5.8 | IC6.7 61.38,52.38 63.5,54.5 63.5,69.96 C9.2 65.92,72.62 IC4.2 | X2.C1 50,91.5 50,97.5 | IC2.7 52.62,72.58 C4.2 50,69.96 50,67.67 50,62.64 50,52.58 50,52 47.81,49.81 IC9.8 | 88,72.5 88,72.69 88,76 | IC4.7 IC4.6 IC4.5 IC4.4 IC4.3 IC4.2 | JP1.3 89,43.79 89,47 97.5,47 | 21,14.5 24,12.5 | 68.5,11.5 71,11.5 | v5.65,16.1 1.5,16.1 1.5,16 | v5.65,11.1 1.5,11.1 1.5,11 | v4.15,32.6 1.5,32.6 1.5,32.5 | v4.15,30.1 1.5,30.1 1.5,29.5
  Bottom 1.5: 1.5,1.5 15.5,1.5 19.5,1.5 45.5,1.5 65,1.5 69,1.5 81.84,1.5 94,1.5 97.5,1.5 97.5,4 97.5,29.26 97.5,47 97.5,76 97.5,97.5 61,97.5 50,97.5 24.5,97.5 1.5,97.5 1.5,95 1.5,93 1.5,74 1.5,69.5 1.5,61.5 1.5,57 1.5,53.5 1.5,32.5 1.5,29.5 1.5,16 1.5,11 1.5,1.5
N$1
  Top 0.254: IC2.1 37.49,76.81 39.78,76.81 IC2.2 | Q1.1 18.52,80.47 23.09,80.47 23.55,80.92 R6.1
  Bottom 0.254: IC2.1 37.26,76.81 27.89,76.81 23.77,80.92 R6.1
N$2
  Top 0.254: IC2.5 47.32,76.81 45.03,76.81 IC2.4 44.81,76.81 42.52,76.81 IC2.3 42.29,76.81 40.69,78.41 31.32,78.41 | 31.32,78.41 31.32,80.92 R6.2 | 31.32,78.41 31.32,75.21 R5.1
N$3  (via drill 0.61)
  Top 0.254: v30.18,48.69 27.66,46.18 27.66,40.01 24.46,36.8 24,36.8 IC1.13 | v41.38,81.84 41.6,81.61 49.61,81.61 52.12,84.12 52.58,84.12 IC2.8
  Bottom 0.254: v30.18,48.69 30.18,50.29 37.95,58.06 41.38,58.06 | 41.38,58.06 45.72,58.06 46.18,57.61 IC9.5 | 41.38,58.06 v41.38,81.84
N$4
  Top 0.254: 7.54,90.3 11.2,90.3 SW2.1 | 7.54,90.3 5.03,90.3 SW2.2 | 7.54,90.3 7.54,82.98 5.49,80.92 4.34,80.92 2.74,79.32 2.74,72.92 4.12,71.55 4.12,69.95 X3.14
N$6
  Top 0.254: Q1.2 18.52,75.44 23.32,75.44 23.55,75.21 R5.2
  Bottom 0.254: IC2.6 50.06,76.81 42.52,84.35 IC2.12 42.29,84.35 40.01,84.35 IC2.13 39.78,84.12 37.72,82.07 23.32,82.07 22.63,81.38 22.63,80.47 23.55,79.55 23.55,75.21 R5.2
N$8
  Top 0.254: IC2.11 45.03,84.35 47.32,84.35 IC2.10 47.55,84.35 50.06,84.35 IC2.9
N$11
  Top 0.254: R7.1 86.87,13.03 86.87,9.37 87.33,8.91 S1.4 87.55,8.91 93.73,8.91 S1.3 | IC1.9 24,46.63 25.6,45.03 25.6,38.63 24.69,37.72 22.86,37.72 22.17,37.03 22.17,11.2 26.75,6.63 80.47,6.63 81.61,7.77 C13.1
  Bottom 0.254: S1.4 87.33,8.69 82.53,8.69 81.84,8 C13.1
N$12
  Top 0.254: Q3.C 88.92,29.26 87.78,30.4 87.78,36.8 R2.2 87.78,37.03 93.73,42.98 93.73,43.43 JP1.1
N$13
  Top 0.254: R3.2 85.5,22.17 85.5,23.09 91.44,29.03 Q3.B
N$15
  Top 0.254: R4.2 85.5,37.03 85.5,37.72 91.21,43.43 JP1.2
N$16
  Top 0.254: R4.1 77.72,36.8 77.72,32.92 81.38,29.26 Q2.B
N$17
  Top 0.254: LED1.A 81.84,15.54 85.72,15.54 86.64,16.46 R8.1
N$19
  Top 0.254: IC3.4 73.15,60.12 73.15,62.41 IC3.3
N$20
  Top 0.254: IC3.1 73.15,67.44 73.15,65.15 IC3.2 73.38,64.92 79.32,58.98 85.27,58.98 86.64,57.61 IC5.5 86.64,57.38 86.64,55.09 IC5.6
N$22
  Top 0.254: IC5.7 86.64,52.58 82.75,52.58 81.61,53.72 77.04,53.72 73.38,57.38 IC3.5
N$23
  Bottom 0.254: IC7.4 59.89,38.41 71.32,49.84 71.32,53.03 73.15,54.86 IC3.6
N$24
  Bottom 0.254: IC6.5 59.66,57.38 56.46,54.18 56.46,44.35 55.78,43.66 55.78,32.23 59.66,28.35 IC7.8
N$27
  Top 0.254: IC8.9 46.41,20.57 51.66,20.57 52.81,21.72 73.84,21.72 74.98,20.57 IC7.14
N$28  (via drill 0.61)
  Top 0.254: v48.23,25.6 47.09,24.46 45.26,24.46 44.35,23.55 44.35,20.34 45.26,19.43 76.12,19.43 76.81,20.12 76.81,21.03 76.58,21.26 76.58,22.4 76.81,22.63 76.81,26.06 75.21,27.66 75.21,28.12 IC7.17
  Bottom 0.254: v48.23,25.6 48.23,27.43 48.46,27.66 48.46,38.63 46.41,40.69 IC8.1
N$29
  Top 0.254: IC7.16 74.98,25.83 72.01,25.83 60.58,37.26 54.86,37.26 53.95,38.18 IC8.19
N$30
  Top 0.254: IC7.15 74.98,23.32 73.84,23.32 62.41,34.75 54.86,34.75 53.95,35.66 IC8.18
N$35  (via drill 0.61)
  Top 0.254: v88.47,60.81 86.87,62.41 IC5.3
  Bottom 0.254: v88.47,60.81 88.47,54.41 87.78,53.72 85.95,53.72 79.78,47.55 79.78,40.92 76.12,37.26 74.07,37.26 66.52,29.72 66.52,27.66 59.89,21.03 59.89,20.57 IC7.11
N$36
  Bottom 0.254: IC7.13 75.21,18.06 82.98,25.83 82.98,42.98 92.58,52.58 92.58,53.26 94.18,54.86 IC5.11
N$37  (via drill 0.61)
  Top 0.254: v70.64,45.03 72.01,45.03 75.67,48.69 95.33,48.69 96.01,49.38 96.01,60.81 94.41,62.41 IC5.14
  Bottom 0.254: v70.64,45.03 65.61,40.01 65.61,31.55 59.89,25.83 IC7.9
N$38  (via drill 0.61)
  Top 0.254: v87.1,45.72 v78.87,45.72
  Bottom 0.254: v78.87,45.72 77.5,47.09 74.07,47.09 66.06,39.09 66.06,29.49 59.89,23.32 IC7.10 | v87.1,45.72 87.1,46.41 91.9,51.21 95.33,51.21 96.01,51.89 96.01,58.29 94.41,59.89 IC5.13
N$39  (via drill 0.61)
  Top 0.254: v75.67,56.46 77.72,56.46 79.78,58.52 81.84,58.52 84.81,55.55 84.81,54.63 85.95,53.49 93.27,53.49 94.18,52.58 IC5.10
  Bottom 0.254: v75.67,56.46 72.47,56.46 70.87,54.86 70.87,51.44 60.35,40.92 59.89,40.92 IC7.3
N$40  (via drill 0.61)
  Top 0.254: v68.81,26.98 65.15,30.63 59.89,30.63 IC7.7
  Bottom 0.254: v68.81,26.98 71.78,26.98 74.52,29.72 76.35,29.72 82.53,35.89 82.53,43.2 92.13,52.81 92.13,55.32 94.18,57.38 IC5.12
N$41
  Top 0.254: IC8.8 46.41,23.32 51.89,23.32 53.03,24.46 54.86,24.46 58.06,27.66 58.06,31.55 59.66,33.15 IC7.6
PA0  (via drill 0.61)
  Top 0.254: v42.29,48.46 40.23,50.52 38.41,50.52 37.26,51.66 37.26,65.15 39.09,66.98 IC1.40 | v41.15,35.2 37.95,35.2 35.89,33.15 35.89,12.8 X1.2
  Bottom 0.254: v42.29,48.46 42.29,36.35 v41.15,35.2
PA1  (via drill 0.61)
  Top 0.254: v21.03,37.95 v21.03,43.66
  Bottom 0.254: v21.03,43.66 21.03,61.27 22.86,63.09 24.46,63.09 25.83,64.47 39.09,64.47 IC1.39 | v21.03,37.95 21.03,37.26 23.09,35.2 24.92,35.2 28.12,32 28.12,23.09 38.41,12.8 X1.3
PA2
  Top 0.254: IC1.38 39.32,61.95 45.26,56.01 47.32,56.01 52.12,51.21 52.12,49.38 56.92,44.58 61.72,44.58 74.52,31.77 76.35,31.77 77.95,30.18 77.95,23.32 78.87,22.4 78.87,19.66 75.67,16.46 53.03,16.46 50.52,13.95 42.52,13.95 41.38,12.8 X1.4
PA3  (via drill 0.61)
  Top 0.254: v35.89,39.78 v29.95,45.72 | v37.26,19.66 37.26,18.52 40.92,14.86 v42.06,14.86
  Bottom 0.254: v29.95,45.72 29.26,46.41 29.26,50.06 38.63,59.44 39.09,59.44 IC1.37 | v35.89,39.78 35.89,21.03 v37.26,19.66 | v42.06,14.86 44.12,12.8 X1.5
PA4
  Bottom 0.254: IC1.36 39.09,56.92 39.09,56.46 37.26,54.63 37.26,54.18 38.41,53.03 40.23,53.03 41.38,51.89 41.38,41.83 39.78,40.23 37.95,40.23 36.35,38.63 36.35,21.95 38.41,19.89 40.23,19.89 46.63,13.49 46.63,12.8 X1.6
PA5
  Bottom 0.254: IC1.35 39.32,54.41 40.23,53.49 40.46,53.49 43.89,50.06 43.89,45.26 49.15,40.01 49.15,21.26 47.09,19.2 45.26,19.2 44.35,18.29 44.35,17.6 49.38,12.57 X1.7
PA6
  Bottom 0.254: IC1.34 39.32,51.66 40.92,50.06 40.92,43.89 39.78,42.75 32.23,42.75 31.55,42.06 31.55,24 42.75,12.8 42.75,12.34 43.43,11.66 51.21,11.66 52.12,12.57 X1.8
PA7  (via drill 0.61)
  Top 0.254: v65.38,69.04 65.38,69.49 61.27,73.61 43.43,73.61 36.8,66.98 36.8,51.44 38.18,50.06 38.41,50.06 39.09,49.38 IC1.33 | v63.32,45.26 68.58,45.26 74.3,39.55 76.58,39.55 82.53,33.6 82.53,22.63 75.89,16 58.29,16 55.09,12.8 X1.9
  Bottom 0.254: v65.38,69.04 65.38,47.32 v63.32,45.26
PB0  (via drill 0.61)
  Top 0.254: v75.21,69.95 75.67,69.95 79.32,66.29 93.04,66.29 94.18,65.15 IC5.15 | v40.46,63.32 45.26,58.52 48.01,58.52 52.81,53.72 v64.47,53.72
  Bottom 0.254: v75.21,69.95 64.92,69.95 64.47,69.49 v64.47,53.72 64.47,48.46 59.89,43.89 59.89,43.43 IC7.2 | v40.46,63.32 40.92,63.78 40.92,64.92 40.23,65.61 38.41,65.61 37.03,66.98 24,66.98 IC1.1
PB2  (via drill 0.61)
  Top 0.254: v22.17,42.98 22.17,37.72 21.26,36.8 v21.26,12.12
  Bottom 0.254: v22.17,42.98 22.17,59.89 23.77,61.49 23.77,61.95 IC1.3 | v21.26,12.12 24.92,8.46 28.8,8.46 32.92,12.57 X1.1
PB3  (via drill 0.61)
  Top 0.254: v28.57,37.26 v28.57,45.72 | v38.41,14.4 40.01,12.8 40.01,12.34 40.69,11.66 59.44,11.66 60.35,12.57 X1.11
  Bottom 0.254: v28.57,45.72 28.57,54.41 24,58.98 24,59.44 IC1.4 | v28.57,37.26 28.57,24.23 v38.41,14.4
PB6
  Top 0.254: IC1.7 24,51.89 24,52.35 36.35,64.69 36.35,67.21 44.12,74.98 61.72,74.98 63.32,76.58 IC4.1
  Bottom 0.254: IC6.2 59.89,65.15 59.89,65.61 62.64,68.35 62.64,72.01 63.55,72.92 63.55,76.58 IC4.1
PB7
  Top 0.254: IC8.3 46.18,35.89 46.18,38.18 IC8.2 46.18,38.41 44.35,40.23 38.41,40.23 37.26,41.38 37.26,42.98 30.63,49.61 29.72,49.61 29.49,49.38 24,49.38 IC1.8
PC0
  Top 0.254: IC1.22 39.09,21.49 37.26,23.32 37.26,31.77 38.18,32.69 44.58,32.69 45.03,32.23 52.35,32.23 53.72,30.86 IC8.16
PC1
  Bottom 0.254: IC1.23 39.32,24 42.29,24 45.26,26.98 47.09,26.98 48.01,27.89 48.01,31.55 46.41,33.15 IC8.4
PC2
  Top 0.254: IC1.24 39.32,26.52 44.81,26.52 45.26,26.98 52.58,26.98 53.72,28.12 IC8.15
PC3
  Top 0.254: IC1.25 39.32,29.03 44.58,29.03 46.18,30.63 IC8.5
PC4
  Top 0.254: IC1.26 39.32,31.77 50.52,31.77 53.03,29.26 54.86,29.26 55.55,28.57 55.55,27.43 53.95,25.83 IC8.14
PC5
  Bottom 0.254: IC8.6 46.18,28.35 45.03,28.35 39.32,34.06 IC1.27
PC6  (via drill 0.61)
  Top 0.254: v48.23,21.95 52.35,21.95 53.72,23.32 IC8.13
  Bottom 0.254: v48.23,21.95 45.26,21.95 44.81,22.4 37.72,22.4 36.8,23.32 36.8,34.75 38.63,36.58 39.09,36.58 IC1.28
PC7
  Bottom 0.254: IC1.29 39.32,39.09 39.32,38.63 40.92,37.03 40.92,36.35 39.78,35.2 37.95,35.2 37.26,34.52 37.26,23.55 37.95,22.86 43.43,22.86 46.18,25.6 IC8.7
PD0  (via drill 0.61)
  Top 0.254: v27.89,14.4 35.2,7.09 73.38,7.09 80.47,14.17 80.47,15.77 85.5,20.8 86.41,20.8 87.55,21.95 R1.1
  Bottom 0.254: v27.89,14.4 26.06,14.4 22.17,18.29 22.17,32 23.77,33.6 23.77,34.06 IC1.14 | Q2.C 78.87,29.03 78.87,24.69 75.89,21.72 74.07,21.72 73.38,21.03 73.38,17.6 74.07,16.92 82.53,16.92 87.55,21.95 R1.1
PD1
  Top 0.254: R3.1 77.5,22.17 77.5,27.89 75.67,29.72 70.64,29.72 60.81,39.55 52.12,39.55 47.32,34.75 43.2,34.75 40.23,37.72 30.4,37.72 24.46,31.77 24,31.77 IC1.15
PD2
  Top 0.254: IC1.16 24,28.8 34.29,18.52 34.29,10.29 X1.14
PD3
  Bottom 0.254: IC1.17 24,26.29 37.26,13.03 37.26,12.34 39.32,10.29 39.78,10.29 X1.16
PD4  (via drill 0.61)
  Top 0.254: v37.72,8 73.61,8 80.01,14.4 80.01,18.75 85.04,23.77 85.04,35.66 76.12,44.58 74.07,44.58 73.38,43.89 73.38,42.52 74.98,40.92 IC7.22
  Bottom 0.254: v37.72,8 35.89,9.83 35.89,10.29 34.52,11.66 34.52,13.26 24,23.77 IC1.18
PD5
  Top 0.254: IC1.19 24,21.26 31.77,13.49 31.77,11.2 34.06,8.91 66.29,8.91 72.92,15.54 76.12,15.54 82.98,22.4 82.98,35.43 75.21,43.2 IC7.23
PD7  (via drill 0.61)
  Top 0.254: v52.12,16.92 45.03,16.92 43.2,18.75 39.32,18.75 IC1.21 | v62.64,73.61 77.72,73.61 80.7,76.58 v80.7,77.95 | v84.81,84.35 v86.64,84.35 | v83.9,86.41 78.18,86.41 76.12,84.35 IC4.9
  Bottom 0.254: v52.12,16.92 54.86,16.92 55.55,17.6 55.55,18.52 54.63,19.43 52.81,19.43 51.44,20.8 51.44,48.46 50.29,49.61 50.29,50.52 50.98,51.21 54.86,51.21 55.55,51.89 55.55,65.61 62.64,72.69 v62.64,73.61 | v80.7,77.95 82.53,77.95 86.64,82.07 v86.64,84.35 | v84.81,84.35 84.81,85.5 v83.9,86.41
PHASE0  (via drill 0.61)
  Top 0.254: v56.92,89.61 41.6,89.61 40.46,88.47 39.55,88.47 X2.C4
  Bottom 0.254: v56.92,89.61 60.35,89.61 62.41,87.55 70.64,87.55 70.87,87.33 | 70.87,87.33 73.38,84.81 73.38,84.35 IC4.10 | 70.87,87.33 73.15,89.61 73.15,90.98 72.69,91.44 66.52,91.44 65.15,92.81 64.47,92.81 X4.2
PHASE1
  Top 0.254: X4.4 66.98,92.81 67.67,92.81 69.04,91.44 75.21,91.44 75.89,90.75 75.89,89.61 76.35,89.15 77.72,89.15 78.41,89.84 78.41,90.98 78.87,91.44 88.01,91.44 88.24,91.21 88.24,89.38 83.67,84.81 80.7,84.81 79.78,83.9 79.78,83.21 78.41,81.84 72.01,81.84 71.09,82.75 71.09,84.12 IC4.11
  Bottom 0.254: X2.C5 37.03,88.47 37.95,88.47 39.09,89.61 42.29,89.61 43.2,88.7 43.2,88.01 44.58,86.64 68.58,86.64 70.87,84.35 IC4.11
PHASE2  (via drill 0.61)
  Top 0.254: v49.15,82.53 42.06,82.53 41.38,83.21 41.38,85.04 40.23,86.18 37.72,86.18 35.66,88.24 34.52,88.24 X2.C6 | v81.15,83.9 78.64,81.38 71.32,81.38 68.58,84.12 IC4.12
  Bottom 0.254: v49.15,82.53 56.01,82.53 59.66,86.18 66.52,86.18 68.35,84.35 IC4.12 | v81.15,83.9 80.7,84.35 80.7,94.64 79.1,96.24 73.38,96.24 70.18,93.04 69.49,93.04 X4.6
PHASE3  (via drill 0.61)
  Top 0.254: v41.83,86.41 41.6,86.64 39.55,86.64 38.41,87.78 38.41,88.47 37.26,89.61 34.06,89.61 32.92,88.47 32,88.47 X2.C7
  Bottom 0.254: v41.83,86.41 44.12,86.41 44.35,86.18 45.26,86.18 46.41,85.04 46.41,83.21 48.01,81.61 54.63,81.61 54.86,81.84 63.55,81.84 65.84,84.12 IC4.13 66.06,84.12 68.35,81.84 73.15,81.84 74.75,83.44 74.75,85.27 75.67,86.18 75.67,90.98 75.21,91.44 74.07,91.44 72.69,92.81 72.01,92.81 X4.8
WP  (via drill 0.61)
  Top 0.254: v72.47,82.75 72.92,82.75 73.15,82.53 77.04,82.53 v77.27,82.75
  Bottom 0.254: v72.47,82.75 72.47,85.04 70.41,87.1 46.63,87.1 45.72,88.01 45.72,90.98 44.58,92.13 44.58,93.27 X2.A2 | X4.20 87.1,92.81 85.72,91.44 85.72,81.84 82.53,78.64 81.38,78.64 80.24,79.78 80.24,84.81 78.87,86.18 78.41,86.18 77.27,85.04 v77.27,82.75 75.89,81.38 55.09,81.38 51.44,77.72 51.44,74.98 44.35,67.89 44.35,67.21 45.03,66.52 46.86,66.52 48.01,65.38 48.01,57.15 47.09,56.24 45.26,56.24 44.35,55.32 44.35,49.38 45.03,48.69 46.18,48.69 50.98,43.89 50.98,20.57 52.58,18.97 52.81,18.97 53.72,18.06 IC8.11
WRITE  (via drill 0.61)
  Top 0.254: v58.98,93.95 60.12,95.1 73.38,95.1 74.52,93.95 74.52,93.04 X4.10 | v51.44,93.95 47.78,93.95 47.32,94.41 40.46,94.41 39.55,93.5 X2.A4 39.32,93.5 38.41,93.5 37.49,94.41 28.8,94.41 27.89,93.5 27.89,68.58 24,64.69 IC1.2 23.77,64.47 22.17,62.87 22.17,51.44 22.86,50.75 30.18,50.75 32.69,48.23 39.78,48.23 40.46,47.55 52.35,47.55 v56.69,43.2
  Bottom 0.254: v51.44,93.95 v58.98,93.95 | v56.69,43.2 56.69,39.32 59.66,36.35 59.66,35.89 IC7.5

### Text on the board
tNames: APPLE FDD | AGAT FDD | Version 1.0 | [RBSC] 2016 | ATX Power Connector | Link2 for 140kb FDD [Agat/Apple] | GND | TX | RX | X6 | 12V | GND | GND | PWR2 | 5V | Optional | X5 | 2716/27C16 / 2732/27C32 | 5V | Install for -12V | for Apple drives | Original Design by Vladimir & Garnizon | ATMEGA 16 | GND | + | GND | Optional | SW1 | Molex Power | Connector | 12V | LPT Port | PWR1 | RESET
bNames: Link2 for 140kb FDD [Agat/Apple] | Version 1.0 | Original Design by Vladimir & Garnizon | [RBSC] 2016 | Copyright (C) 2010-2016 | Schematics and Board by Wierzbowsky [RBSC]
